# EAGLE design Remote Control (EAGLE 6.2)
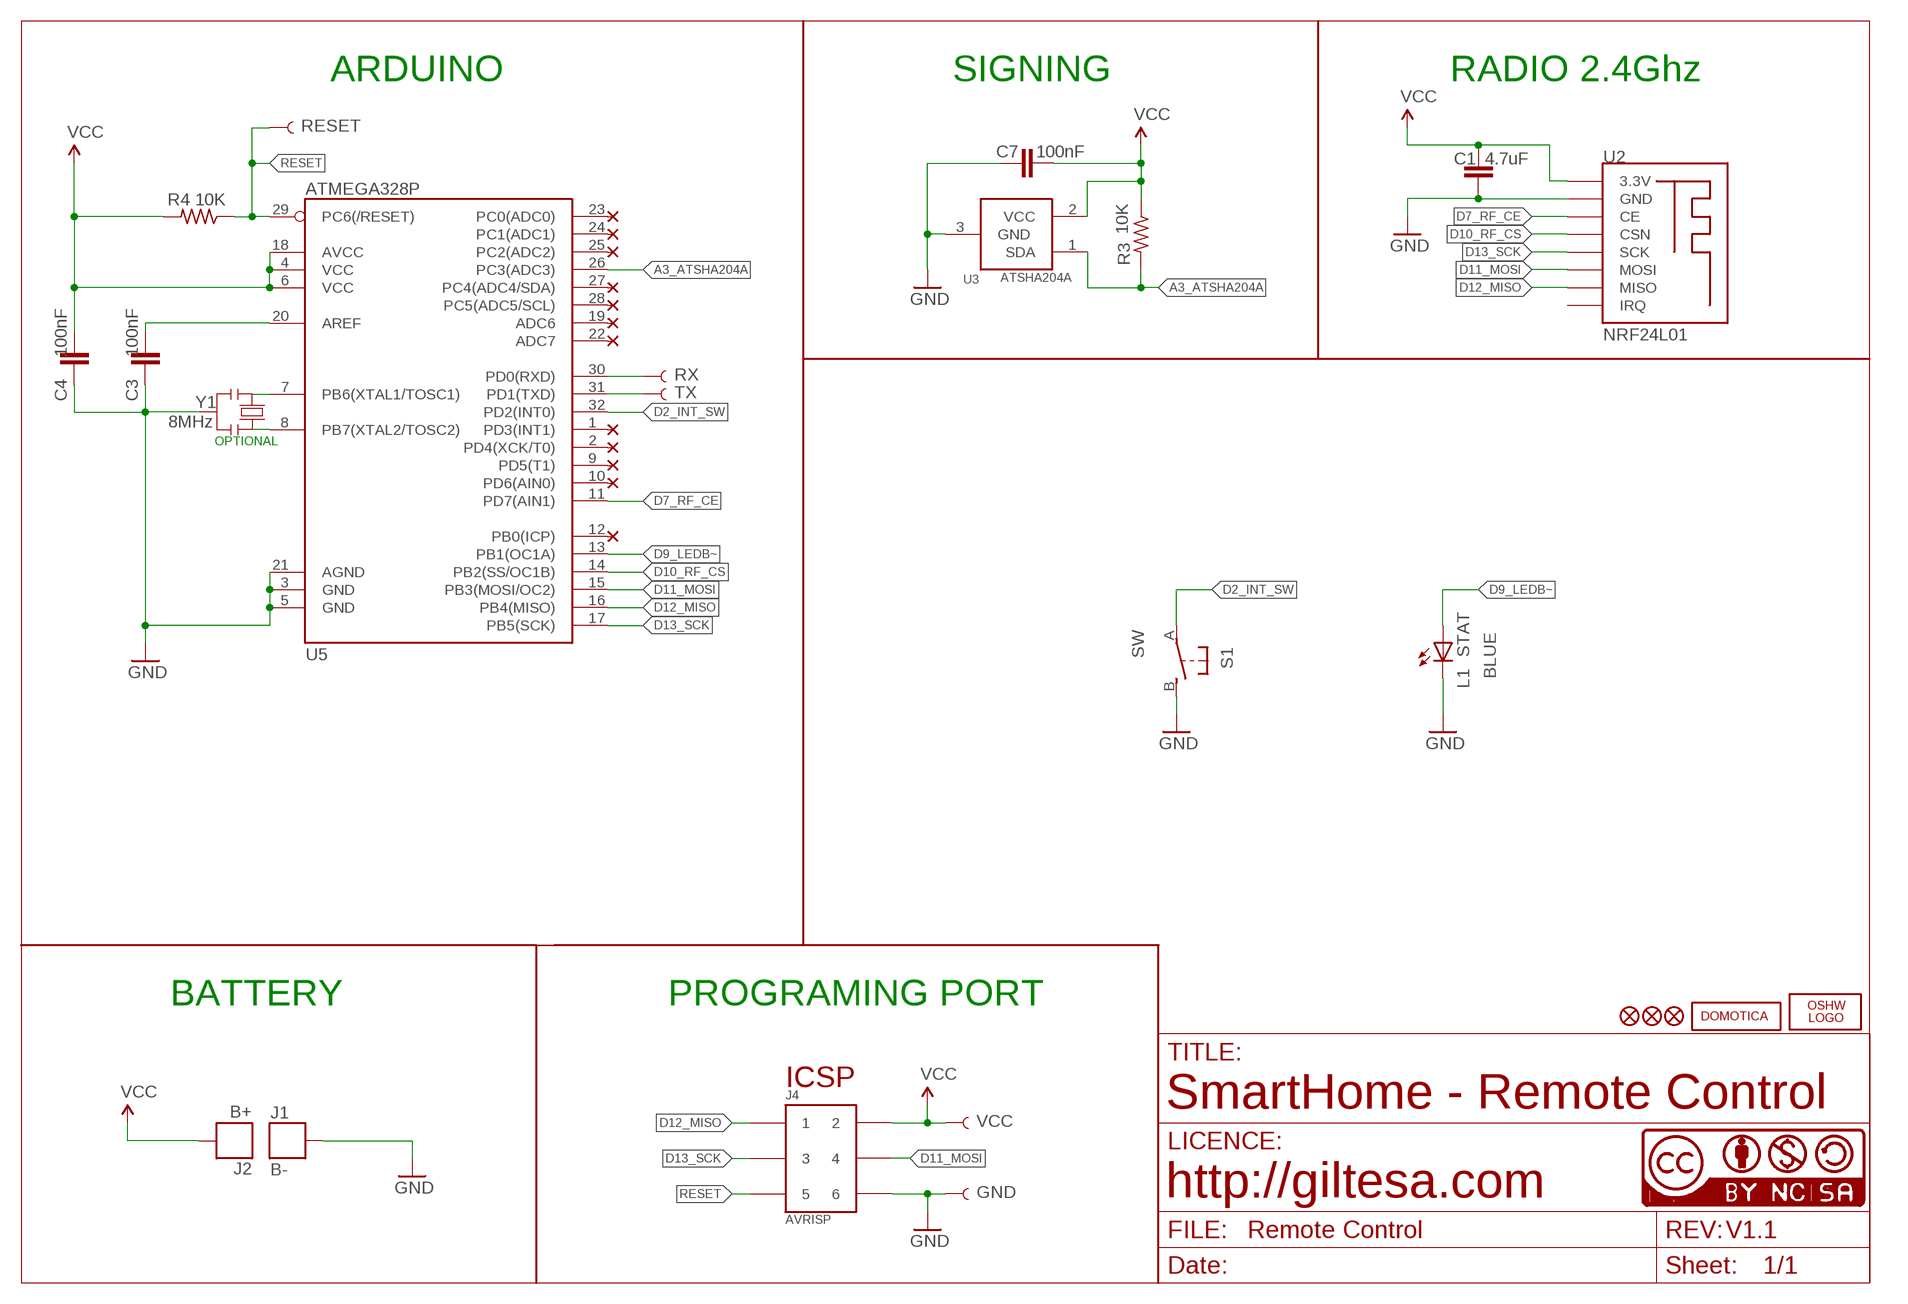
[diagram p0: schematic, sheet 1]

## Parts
C1  4.7uF  C1206  [C1206]
C3  100nF  C0603  [C0603]
C4  100nF  C0603  [C0603]
C7  100nF  C0603  [C0603]
J1  B-  PAD_KEYFINDER  [PAD_KEYFINDER]
J2  B+  PAD_KEYFINDER  [PAD_KEYFINDER]
J4  AVRISP  HEAD3X2  [HEAD3X2]
L1  STAT  LEDCHIP-LED0805  [CHIP-LED0805]
LOGO1  OSHW_LOGO_FILLX0150-NT  [OSHW_FILLX150_NOTEXT]
R3  10K  R0603  [R0603]
R4  10K  R0603  [R0603]
S1  SW  SWITCH_2P  [SWITCH-5X5MM-SMD]
TP1  RX  TEST-POINT3X4  [PAD.03X.04]
TP2  TX  TEST-POINT3X4  [PAD.03X.04]
TP3  RESET  TEST-POINT3X4  [PAD.03X.04]
TP4  VCC  TEST-POINT3X4  [PAD.03X.04]
TP5  GND  TEST-POINT3X4  [PAD.03X.04]
U2  NRF24L01  NRF24L01_SMD  [NRF24L01_SMD]
U3  ATSHA204A  IC_ATSHA204A_CRYPT  [SOT23-3]
U5  ATMEGA328P  ATMEGA328_2  [MLF32_HAND_SOLDERING]
U$5  DOMOTICA10MM  [DOMOTICA-10MM]
U$6  FIDUCIAL1X2  [FIDUCIAL-1X2]
U$7  FIDUCIAL1X2  [FIDUCIAL-1X2]
U$14  FIDUCIAL1X2  [FIDUCIAL-1X2]
U$15  CC-NC-BCNIX  [CC-NC-B_NIX]
Y1  8MHz  RESONATORMU  [RESONATOR]

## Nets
A3_ATSHA204A: R3.2 U3.1(SDA) U5.26(PC3(ADC3))
D2_INT_SW: S1.A U5.32(PD2(INT0))
D7_RF_CE: U2.CE U5.11(PD7(AIN1))
D9_LEDB~: L1.A U5.13(PB1(OC1A))
D10_RF_CS: U2.CSN U5.14(PB2(SS/OC1B))
D11_MOSI: J4.4 U2.MOSI U5.15(PB3(MOSI/OC2))
D12_MISO: J4.1 U2.MISO U5.16(PB4(MISO))
D13_SCK: J4.3 U2.SCK U5.17(PB5(SCK))
GND [gnd]: C1.2 C3.1 C4.1 C7.1 J1.P$2 J4.6 L1.C S1.B TP5.P$1 U2.GND U3.3(GND) U5.3(GND) U5.5(GND) U5.21(AGND) Y1.2
N$1: TP1.P$1 U5.30(PD0(RXD))
N$2: TP2.P$1 U5.31(PD1(TXD))
N$29: U5.7(PB6(XTAL1/TOSC1)) Y1.1
N$30: U5.8(PB7(XTAL2/TOSC2)) Y1.3
N$33: C3.2 U5.20(AREF)
RESET: J4.5 R4.1 TP3.P$1 U5.29(PC6(/RESET))
VCC: C1.1 C4.2 C7.2 J2.P$2 J4.2 R3.1 R4.2 TP4.P$1 U2.3.3V U3.2(VCC) U5.4(VCC) U5.6(VCC) U5.18(AVCC)
Unconnected: U2.IRQ U5.1(PD3(INT1)) U5.2(PD4(XCK/T0)) U5.9(PD5(T1)) U5.10(PD6(AIN0)) U5.12(PB0(ICP)) U5.19(ADC6) U5.22(ADC7) U5.23(PC0(ADC0)) U5.24(PC1(ADC1)) U5.25(PC2(ADC2)) U5.27(PC4(ADC4/SDA)) U5.28(PC5(ADC5/SCL))

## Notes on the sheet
- ARDUINO | SIGNING | RADIO 2.4Ghz
- OPTIONAL
- BLUE
- BATTERY | PROGRAMING PORT
- ICSP
- SmartHome - Remote Control
- http://giltesa.com
- V1.1

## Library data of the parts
C1 = ,giltesa:C1206
C3 C4 C7 = ,giltesa:C0603
J1 J2 = ,giltesa:PAD_KEYFINDER
J4 = MyCON2:HEAD3X2
L1 = led:LED: LED
LOGO1 = ohw-logo:OSHW_LOGO_FILL
R3 R4 = ,giltesa:R0603
S1 = ,giltesa:SWITCH_2P
TP1-TP5 = SparkFun-Connectors:TEST-POINT: SparkFun Test Points
U2 = ,giltesa:NRF24L01_SMD
U3 = TD-MySensors:IC_ATSHA204A_CRYPT
U5 = ,giltesa:ATMEGA328
U$5 = ,giltesa_logos:DOMOTICA
U$6 U$7 U$14 = SparkFun:FIDUCIAL: Fiducial Alignment Points
U$15 = cc-by-nc-sa:CC-NC-BC: All hardware is licensed under the Creative Commons
Y1 = MySMD2:RESONATOR

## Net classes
2 gnd: width 0.305 mm, drill 0.406 mm, clearance 0.203 mm
3 usbvcc: width 0.203 mm, drill 0.406 mm, clearance 0.203 mm
4 USBpair: width 0.254 mm, drill 0.406 mm, clearance 0.61 mm

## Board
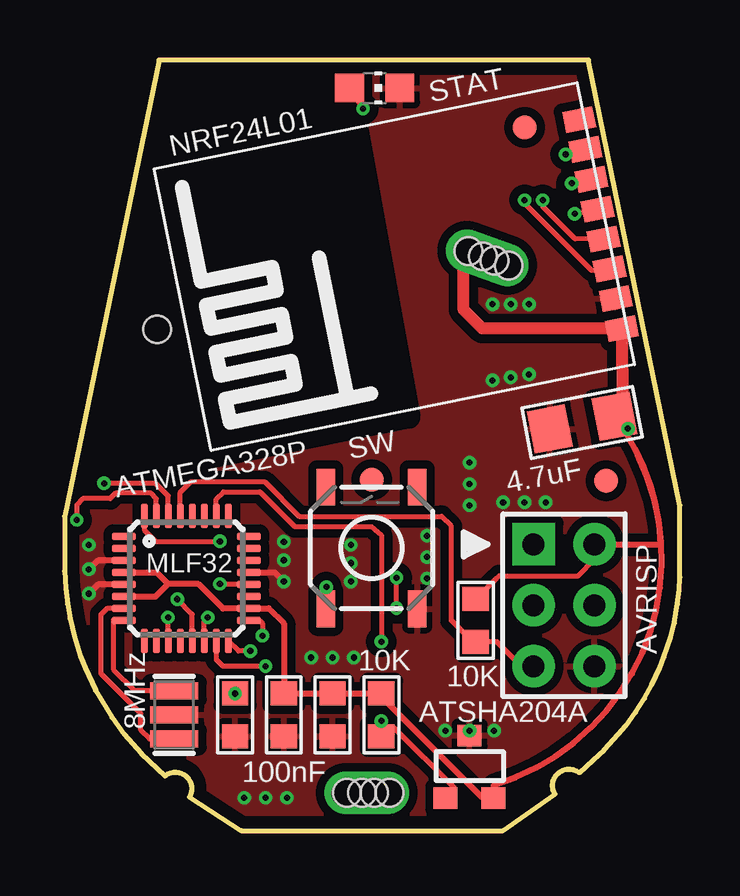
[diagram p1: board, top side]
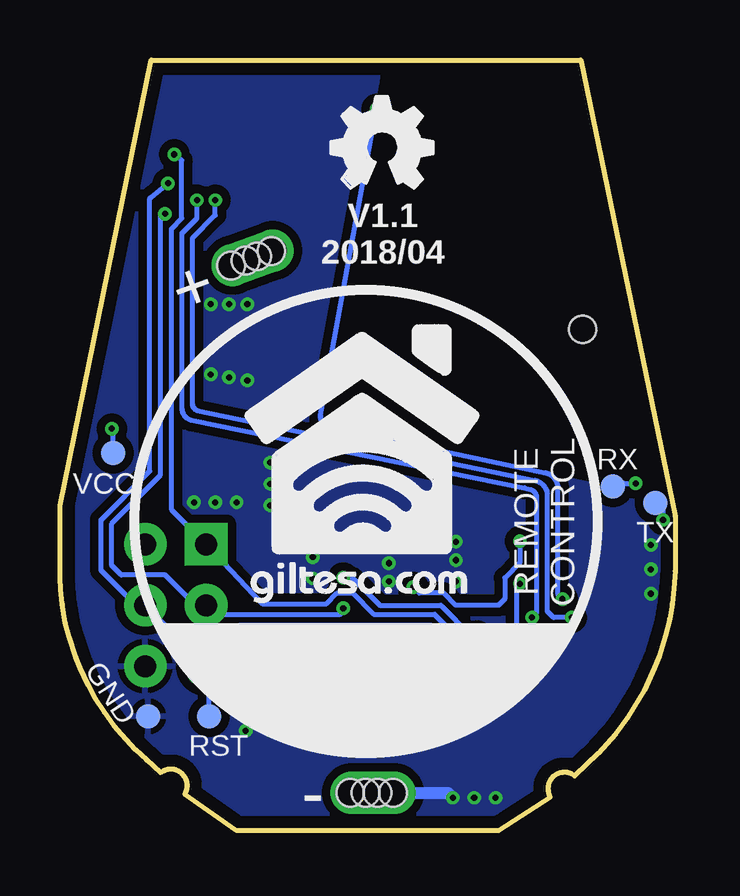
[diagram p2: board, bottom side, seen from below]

Size 25.65 x 32.13 mm. Coordinates in mm from the lower left corner, seen from the top.
Outline: 7.37,0 18.29,0 20.45,1.52 arc-160 21.46,2.41 22.05,2.95 22.5,3.38 23.09,4.01 23.39,4.37 23.8,4.93 24.18,5.51 24.49,6.07 24.82,6.78 24.99,7.24 25.27,8.08 25.43,8.66 25.55,9.45 25.63,10.03 25.65,10.57 25.65,13.56 21.84,32.13 3.94,32.13 0,13.11 0,10.82 0.05,10.11 0.13,9.45 0.23,8.84 0.41,8.13 0.66,7.29 0.86,6.78 1.29,5.84 1.98,4.72 2.49,4.01 3.2,3.23 4.19,2.29 arc-160 5.21,1.4 7.37,0
Copper layers (1*16): Top 0.035mm / dielectric 1.6mm / Bottom 0.035mm
Design rules: minimum track width 6mil, minimum drill 12mil, track to track 6mil, track to pad 6mil, pad to pad 6mil, via to via 8mil, smd to smd 0mil, copper to edge 20mil, drill to drill 10mil, minimum pad ring 6mil, minimum via ring 6mil, stop-mask expansion 0mil, vias tented up to drill 100mil, thermal gap 10mil
Holes 1.14 mm at 3.86,20.9
tRestrict: 4 lines
bRestrict: 4 lines

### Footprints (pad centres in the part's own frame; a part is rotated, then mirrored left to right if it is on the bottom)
C1206 = smd 1.6 x 1.8: 1 -1.362,0; 2 1.387,0
C0603 = smd 1 x 1.1: 1 -0.901,0; 2 0.901,0
PAD_KEYFINDER = drill 1.143 pad 1.778 offset: P$2 -0.889,0; P$3 0.889,0 | hole 1.143: -0.191,0; 0.318,0; -0.826,0; 0.953,0
HEAD3X2 = drill 0.914 pad 1.778 square: 1 0,0 | drill 0.914 pad 1.778: 2 0,2.54; 3 2.54,0; 4 2.54,2.54; 5 5.08,0; 6 5.08,2.54
CHIP-LED0805 = smd 1.2 x 1.2: A 0,-1.05; C 0,1.05
R0603 = smd 1 x 1.1: 1 -0.901,0; 2 0.901,0
SWITCH-5X5MM-SMD = smd 1.524 x 0.762: A -2.54,1.905; B -2.54,-1.905; NC@1 2.54,1.905; NC@2 2.54,-1.905
PAD.03X.04 = smd 1.016 x 1.016: P$1 0,0
NRF24L01_SMD = smd 0.9 x 1.27: 3.3V 1.575,0.203; CE 4.115,0.203; CSN 5.385,0.203; GND 2.845,0.203; IRQ 10.465,0.203; MISO 9.195,0.203; MOSI 7.925,0.203; SCK 6.655,0.203
SOT23-3 = smd 1 x 0.9: 1 -1,-1.3; 2 1,-1.3; 3 0,1.3
MLF32_HAND_SOLDERING = smd 1.016 x 0.3: 1 -2.604,1.75; 2 -2.604,1.25; 3 -2.604,0.75; 4 -2.604,0.25; 5 -2.604,-0.25; 6 -2.604,-0.75; 7 -2.604,-1.25; 8 -2.604,-1.75; 17 2.604,-1.75; 18 2.604,-1.25; 19 2.604,-0.75; 20 2.604,-0.25; 21 2.604,0.25; 22 2.604,0.75; 23 2.604,1.25; 24 2.604,1.75 | smd 0.3 x 1.016: 9 -1.75,-2.604; 10 -1.25,-2.604; 11 -0.75,-2.604; 12 -0.25,-2.604; 13 0.25,-2.604; 14 0.75,-2.604; 15 1.25,-2.604; 16 1.75,-2.604; 25 1.75,2.604; 26 1.25,2.604; 27 0.75,2.604; 28 0.25,2.604; 29 -0.25,2.604; 30 -0.75,2.604; 31 -1.25,2.604; 32 -1.75,2.604
FIDUCIAL-1X2 = smd 1 x 1: 1 0,0
RESONATOR = smd 0.7 x 2: 1 -1,0; 2 0,0; 3 1,0

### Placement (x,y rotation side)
C1  21.59,17.02 191 top
C3  7.11,4.83 90 top
C4  9.14,4.83 90 top
C7  11.18,4.83 90 top
J1  12.6,1.57 0 top
J2  17.62,23.88 340 top
J4  19.56,11.94 270 top
L1  12.93,30.96 270 top
LOGO1  14.35,26.8 0 bottom
R3  13.21,4.83 270 top
R4  17.14,8.76 90 top
S1  12.8,11.79 90 top
TP1  2.6,14.35 0 bottom
TP2  0.83,13.65 0 bottom
TP3  19.43,4.76 0 bottom
TP4  23.43,15.75 0 bottom
TP5  21.97,4.76 0 bottom
U2  23.75,19.43 101.5 top
U3  16.89,2.67 0 top
U5  5.08,10.52 0 top
U$5  18.03,9.4 0 bottom
U$6  12.8,14.63 0 top
U$7  19.18,29.31 0 top
U$14  22.58,14.58 0 top
U$15  0,0 0 top
Y1  4.57,4.83 90 top

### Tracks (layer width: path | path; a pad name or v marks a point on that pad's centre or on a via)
A3_ATSHA204A  (via drill 0.25)
  Top 0.203: U5.26 6.33,13.82 6.63,14.12 8.15,14.12 9.6,12.68 12.8,12.68 13.21,12.32 v13.21,7.87 | U3.1 16.26,1.73 16.26,1.78 13.72,4.32 13.34,4.32 v13.21,4.57 R3.2
  Bottom 0.203: v13.21,7.87 v13.21,4.57
D2_INT_SW  (via drill 0.25)
  Top 0.203: U5.32 3.33,12.54 3.81,12.06 v6.48,12.06 | S1.A 10.9,10.13 v10.92,10.16
  Bottom 0.203: v10.92,10.16 10.67,9.91 9.65,9.91 9.14,9.4 7.37,9.4 7.11,9.65 7.11,10.54 6.48,11.18 v6.48,12.06
D7_RF_CE  (via drill 0.25)
  Top 0.203: U5.11 4.33,8.88 v4.32,8.89 | v19.18,26.29 19.18,26.16 21.97,23.37 22.7,23.37 U2.CE
  Bottom 0.203: v4.32,8.89 5.08,8.89 5.33,9.14 5.33,14.03 arc-70 5.84,14.61 19.94,17.53 arc70 20.13,17.78 20.13,24.7 19.18,25.65 v19.18,26.29
D9_LEDB~  (via drill 0.25)
  Top 0.203: v12.45,30.1 L1.A | U5.13 5.33,9.02 v4.7,9.65
  Bottom 0.203: v12.45,30.1 14.8,17.34 arc-90 14.41,16.83 5.4,14.92 arc70 4.89,14.29 4.89,9.84 v4.7,9.65
D10_RF_CS  (via drill 0.25)
  Top 0.203: 22.31,24.89 22.31,24.72 | 22.31,24.72 22.1,24.51 | U5.14 5.83,8.75 v5.97,8.89 | v19.94,26.29 19.94,26.02 21.28,24.68 U2.CSN 22.48,24.72 22.31,24.72
  Bottom 0.203: v5.97,8.89 5.78,9.08 5.78,13.91 arc-70 6.03,14.22 6.29,14.29 20.19,17.12 arc70 20.57,17.59 20.57,24.89 19.94,25.53 v19.94,26.29
D11_MOSI  (via drill 0.25)
  Top 0.203: 22.1,27.18 22.1,27.11 U2.MOSI v21.14,26.99 | v8.38,6.86 6.6,6.86 6.33,7.13 U5.15
  Bottom 0.203: v21.14,26.99 21.84,26.42 21.91,26.35 21.91,14.99 23.94,12.95 23.94,10.86 22.48,9.4 J4.4 20.83,8.13 18.61,8.13 18.16,8.57 10.22,8.57 8.51,6.86 v8.38,6.86
D12_MISO  (via drill 0.25)
  Top 0.203: v20.89,28.19 U2.MISO | v7.75,7.49 7.25,7.49 U5.16
  Bottom 0.203: v20.89,28.19 20.57,27.94 20.57,25.53 21.02,25.08 21.02,13.4 J4.1 19.18,11.56 17.21,9.46 14.54,9.46 14.1,9.91 13.46,9.91 12.57,9.02 10.03,9.02 8.51,7.49 v7.75,7.49
D13_SCK  (via drill 0.25)
  Top 0.203: v21.27,25.72 U2.SCK | v13.84,9.27 v13.84,10.54 | U5.17 8.12,8.77 8.26,8.64 v8.26,8.13
  Bottom 0.203: v21.27,25.72 21.46,25.59 21.46,14.83 23.5,12.8 23.5,11.05 23.1,10.65 21.26,10.65 20,9.4 J4.3 19.18,9.02 13.97,9.02 13.84,9.14 v13.84,9.27 | v13.84,10.54 13.46,10.54 12.32,9.4 9.78,9.4 8.51,8.13 v8.26,8.13
GND  (via drill 0.25)
  Top 0.254: U5.21 8.77,10.77 v9.14,10.39 | U5.5 1.4,10.27 v1.02,9.88 | U5.3 1.39,11.27 v1.02,10.9
  Bottom 0.406: 12.54,1.57 J1.P$2 11.65,1.57
  Bottom 0.508: 11.65,1.57 9.47,1.57 v9.27,1.37
  other vias: 7.49,1.37 8.38,1.37 1.02,11.91 15.11,10.52 15.11,11.4 15.11,12.29 19.37,19.02 18.61,18.9 17.84,18.77 17.84,21.95 18.61,21.95 19.37,21.95 9.14,12.04 9.14,11.28 16.89,15.34 16.89,14.45 16.89,13.56 20.07,13.69 19.18,13.69 18.29,13.69 11.94,11.91 11.94,11.15 11.94,10.39 16.89,4.17 15.88,4.17 17.91,4.17 11.18,7.21 10.29,7.21 12.06,7.21
  pour Bottom (isolate 0.356): 25.4,33.02 0,33.02 0,0 25.4,0
  pour Top (isolate 0.356): 0,33.02 25.4,33.02 25.4,0 0,0
N$1  (via drill 0.25)
  Top 0.203: U5.30 4.33,13.96 3.81,14.48 v1.65,14.48
  Bottom 0.203: TP1.P$1 2.29,14.35 2.16,14.48 v1.65,14.48
N$2  (via drill 0.25)
  Top 0.203: U5.31 3.83,13.85 3.61,14.07 2.13,14.07 1.91,13.84 0.76,13.84 0.51,13.59 v0.51,12.95
  Bottom 0.203: 0.89,13.59 TP2.P$1 0.51,13.34 v0.51,12.95
N$29
  Top 0.203: Y1.1 3.54,3.83 3.17,4.19 3.17,4.89 1.52,6.54 1.52,9.02 1.77,9.27 U5.7
N$30
  Top 0.203: Y1.3 4.68,5.84 2.92,5.84 2.03,6.73 2.03,8.8 2.1,8.77 U5.8
N$33  (via drill 0.25)
  Top 0.203: C3.2 v7.11,5.71 | v6.48,10.29 6.5,10.27 U5.20
  Bottom 0.203: v7.11,5.71 6.35,6.48 6.35,8.26 6.6,8.51 6.6,10.16 v6.48,10.29
RESET
  Top 0.203: J4.5 19.05,6.86 18.03,7.87 17.03,7.87 R4.1 17.03,7.86 16.13,8.76 16.13,12.7 15.72,13.11 9.78,13.11 8.33,14.55 5.28,14.55 4.83,14.1 U5.29
  Bottom 0.203: TP3.P$1 19.43,6.73 J4.5
VCC  (via drill 0.25)
  Top 0.203: R4.2 18.03,10.54 18.12,10.63 21.43,10.63 22.1,11.3 J4.2 | v23.5,16.76 23.45,16.76 C1.1
  Top 0.254: U3.2 17.91,1.91 arc110 C1.1 arc-35 24.86,11.94 J4.2 | 16.73,24.2 16.76,24.2 J2.P$2 | 9.26,5.73 9.39,5.73 | 9.39,5.73 9.4,5.71 | 4.32,10.29 5.59,10.29 6.61,9.27 U5.18 8.51,9.27 9.14,8.64 9.14,5.84 9.26,5.73 | 4.32,10.29 3.8,9.77 U5.6 | U5.4 3.84,10.77 4.32,10.29 | C4.2 9.26,5.73 | U3.2 17.56,1.37 | U3.2 17.86,1.4 17.4,1.4 13.34,5.46 13.34,5.6 R3.1 | 9.39,5.73 C7.2 R3.1 | 13.22,5.71 R3.1
  Top 0.406: 17.56,23.9 16.73,23.9 16.73,24.2
  Top 0.508: C1.1 arc90 23.25,17.61 U2.3.3V 17.42,20.94 16.64,21.72 16.64,24.12 16.73,24.2
  Bottom 0.203: TP4.P$1 23.43,16.7 v23.5,16.76

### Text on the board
tPlace: MLF32
bPlace: V1.1 | 2018/04 | + | RX | VCC | CONTROL | REMOTE | TX | GND | RST | -
Document: The PCB has to be manufactured with 1mm thickness.

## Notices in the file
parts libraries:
SparkFun-Connectors: Licensing: Creative Commons ShareAlike 4.0 International - https://creativecommons.org/licenses/by-sa/4.0
